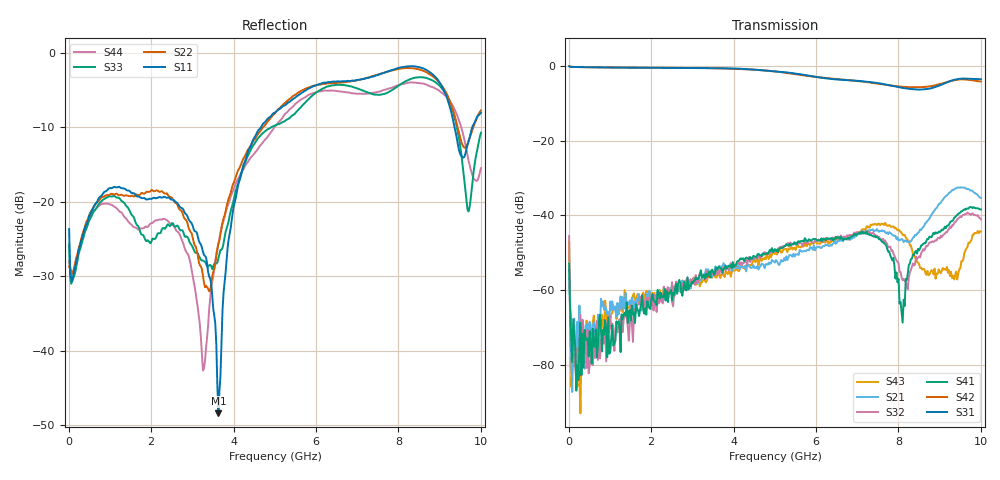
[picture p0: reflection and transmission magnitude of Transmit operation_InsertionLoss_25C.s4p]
! Device:  ADRF5545A
! Description: Dual-Channel, Receiver Front End
! Frequency:  2.4 -  4.2 GHz
! Ports:
!	ANT-CHA	= Port 1
!	ANT-CHB	= Port 2
!  TXOUT-CHA = Port 3
!	TXOUT-CHB = Port 4
! VDD1-CHA, VDD1-CHB, VDD2-CHA, VDD2-CHB, and SWVDD-CHAB = 5 V
! SWCTRL-CHAB = 5 V,  PD-CHAB = 5 V,BP-CHA=BP-CHB=0V
! Temp=25C
! Data:  Data was collected using a calibrated 4 port network analyzer and de-embedded using AtaiTec's In Situ De-Embedding.
! Note:  Analog Devices supplies this data as a sample of measured data
!  for this product.  Your particular data for this product may vary.
!  Data was taken at 25 degrees C.
!  Analog Devices reserves the right to change this data at anytime.
!Correction: S11(Full 4 Port(1,2,3,4))
!S12(Full 4 Port(1,2,3,4))
!S13(Full 4 Port(1,2,3,4))
!S14(Full 4 Port(1,2,3,4))
!S21(Full 4 Port(1,2,3,4))
!S22(Full 4 Port(1,2,3,4))
!S23(Full 4 Port(1,2,3,4))
!S24(Full 4 Port(1,2,3,4))
!S31(Full 4 Port(1,2,3,4))
!S32(Full 4 Port(1,2,3,4))
!S33(Full 4 Port(1,2,3,4))
!S34(Full 4 Port(1,2,3,4))
!S41(Full 4 Port(1,2,3,4))
!S42(Full 4 Port(1,2,3,4))
!S43(Full 4 Port(1,2,3,4))
!S44(Full 4 Port(1,2,3,4))
!S4P File: Measurements: <S11,S12,S13,S14>,
!<S21,S22,S23,S24>,
!<S31,S32,S33,S34>,
!<S41,S42,S43,S44>:
# Hz S  dB  R 50
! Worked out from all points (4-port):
!   401 points, 10 MHz to 10 GHz, reference 50 ohm
!   strongest paths, dB at 10 MHz, 2.507 GHz, 5.005 GHz, 7.503 GHz, 10 GHz:
!     S31: -0.2, -0.6, -1.5, -4.7, -3.6
!     S42: -0.1, -0.6, -1.5, -4.8, -4.2
!     S41: -52.9, -62.7, -49.0, -45.9, -38.4
!     S32: -45.5, -57.9, -49.5, -45.7, -41.0
!     S21: -54.5, -63.0, -52.6, -44.1, -35.3
!     S43: -47.1, -60.8, -50.3, -42.3, -44.3
!   lowest |S11| = -48.4 dB at 3.631 GHz (marker M1), VSWR 1.01, Z = 49.6 + j0.0814 ohm
!   |S11| at or under -10 dB: start of sweep to 4.666 GHz; 9.361 GHz to 9.792 GHz (430.7 MHz wide, 4.5 % of centre)
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1e7  -23.68 -87.1  -40.09 -160.3  -0.14 -3.2  -37.29 -0.5
     -54.54 49.3  -28.70 -113.0  -43.88 169.6  -0.16 -2.7
     -0.16 -2.8  -45.53 -2.7  -25.75 -61.0  -45.63 -80.8
     -52.91 -43.1  -0.12 -2.5  -47.11 -62.1  -27.94 -102.6
2.098e8  -27.63 -71.8  -71.53 102.0  -0.37 -4.8  -87.18 75.4
         -68.41 80.4  -27.08 -73.8  -75.74 -65.7  -0.36 -4.6
         -0.36 -4.8  -75.39 148.8  -28.00 -75.2  -71.89 164.0
         -80.02 79.4  -0.36 -4.6  -85.72 -54.3  -27.08 -73.9
2.582425e9  -19.96 -42.6  -60.58 68.1  -0.58 -56.8  -59.96 -147.6
            -61.23 71.6  -20.14 -57.1  -58.31 -147.2  -0.59 -54.9
            -0.58 -56.7  -59.11 -149.7  -23.37 103.3  -60.15 -9.1
            -59.41 -147.5  -0.59 -54.9  -58.93 -8.5  -23.54 134.8
3.631375e9  -48.38 167.6  -53.88 64.3  -0.66 -81.0  -53.32 -178.1
            -54.57 66.2  -25.62 25.0  -55.18 -176.6  -0.69 -79.0
            -0.65 -81.0  -54.53 170.8  -27.58 -133.4  -56.00 -57.4
            -53.75 -175.6  -0.69 -79.0  -54.74 -53.9  -25.72 -41.6
4.8052e9  -9.00 36.6  -52.69 50.0  -1.34 -111.9  -49.74 140.1
          -53.04 49.8  -9.41 43.7  -50.38 139.3  -1.30 -109.9
          -1.33 -111.9  -50.01 137.1  -10.36 -87.3  -50.20 -147.3
          -50.15 137.7  -1.31 -109.9  -50.49 -141.4  -11.44 -92.8
8.1019e9  -1.94 51.1  -47.26 -43.3  -5.93 176.4  -68.40 31.9
          -46.47 -42.2  -2.10 53.9  -56.23 -26.9  -5.62 -177.1
          -5.93 176.4  -57.34 -17.7  -4.07 103.5  -45.08 -147.9
          -68.66 25.3  -5.61 -177.1  -45.17 -146.7  -4.23 118.0
1e10  -8.07 -171.1  -35.46 151.2  -3.61 113.4  -38.52 -97.3
      -35.31 150.8  -7.75 -174.6  -40.75 -104.3  -4.24 118.7
      -3.60 113.5  -41.04 -108.0  -10.74 -74.4  -43.86 -3.9
      -38.45 -94.8  -4.24 118.7  -44.32 -3.0  -15.51 -45.4
